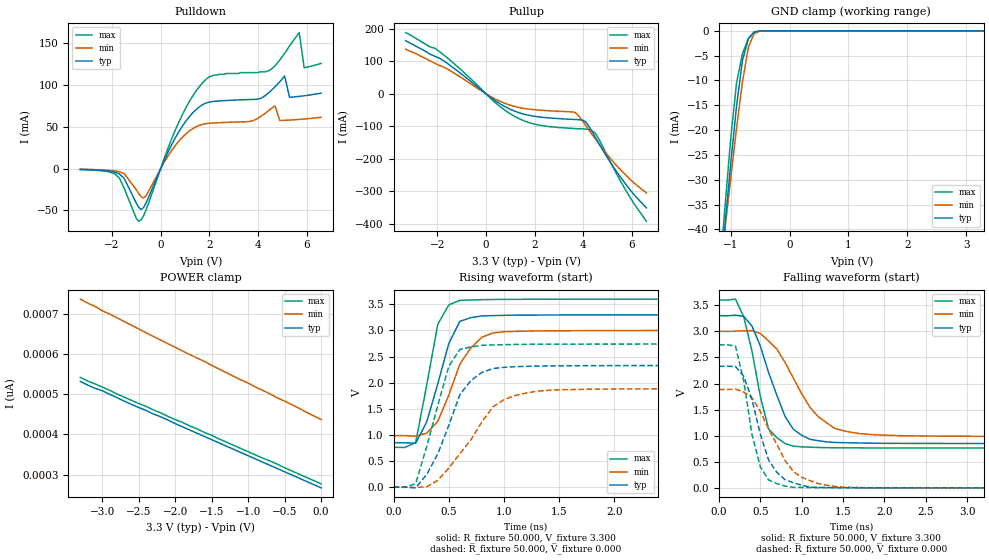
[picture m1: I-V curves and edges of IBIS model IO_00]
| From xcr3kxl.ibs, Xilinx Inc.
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|   Model IO_00
[Model]   IO_00
Model_type   I/O
Polarity   Inverting
Enable   Active-High
Vinl =   0.800V
Vinh =   2.000V
Vmeas =   1.650V
Cref =  50.000pF
Rref =   1.000M
Vref =  0.000V
C_comp   1.250pF   1.000pF   1.500pF
[Temperature Range]   50.000   100.000   0.000
[Voltage Range]   3.300V   3.000V   3.600V
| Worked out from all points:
|   slope of the pulldown table from 0 to 0.495 V, typ, clamps not added: 16 ohm
|   slope of the pullup table from 0 to 0.495 V, typ, clamps not added: 18.3 ohm
|   GND clamp passes 1 mA (typ) near -0.65 V on its own axis
|   rising waveform, R_fixture 50.000, V_fixture 3.300: 20-80 % time 202ps typ, 251ps min, 149ps max; typ from 0.851 V to 3.3 V
|   rising waveform, R_fixture 50.000, V_fixture 0.000: 20-80 % time 278ps typ, 386ps min, 216ps max; typ from 0 V to 2.33 V
|   falling waveform, R_fixture 50.000, V_fixture 3.300: 20-80 % time 334ps typ, 462ps min, 231ps max; typ from 3.3 V to 0.851 V
|   falling waveform, R_fixture 50.000, V_fixture 0.000: 20-80 % time 267ps typ, 385ps min, 199ps max; typ from 2.33 V to 0 V
[Pulldown]
| voltage   I(typ)   I(min)   I(max)
-3.3V     -800uA     -600uA     -1.1mA
-1.7V     -6.1mA     -3.7mA     -11mA
-900mV    -46.35mA   -29.77mA   -62.96mA
-600mV    -41.06mA   -32.32mA   -49.47mA
800mV     46.65mA    34.66mA    59.01mA
1.9V      79mA       54.02mA    108mA
4.5V      92.31mA    70.92mA    118mA
5.1V      111mA      57.94mA    138mA
5.3V      85.46mA    58.26mA    147mA
5.7V      86.62mA    59.04mA    163mA
5.9V      87.32mA    59.5mA     121mA
6.6V      90.4mA     61.49mA    126mA
[Pullup]
| voltage   I(typ)   I(min)   I(max)
-3.3V     163mA      137mA      188mA
-1.9V     109mA      86.62mA    129mA
300mV     -17.18mA   -13mA      -21.73mA
1.2V      -53.91mA   -39.46mA   -70.33mA
2.1V      -70.35mA   -49.69mA   -95.08mA
3.6V      -78.94mA   -56.27mA   -107mA
3.8V      -79.64mA   -66.55mA   -108mA
4.1V      -86.5mA    -97.21mA   -109mA
4.5V      -134mA     -139mA     -121mA
5.5V      -253mA     -231mA     -264mA
6.1V      -311mA     -275mA     -339mA
6.6V      -351mA     -305mA     -392mA
[GND_clamp]
| voltage   I(typ)   I(min)   I(max)
-3.3V     -265mA     -226mA     -304mA
-1.2V     -52.28mA   -50.76mA   -50.82mA
-1.1V     -39.47mA   -40.24mA   -35.9mA
-1V       -26.88mA   -29.77mA   -21.76mA
-900mV    -15.13mA   -19.6mA    -10.45mA
-800mV    -5.967mA   -10.29mA   -4.628mA
-700mV    -1.62mA    -3.333mA   -1.533mA
-600mV    -271uA     -529uA     -194uA
-500mV    -24.86uA   -57.89uA   -10.46uA
-400mV    -1.648uA   -5.395uA   -366nA
3.3V      234pA      465pA      222pA
[POWER_clamp]
| voltage   I(typ)   I(min)   I(max)
-3.3V     532pA      737pA      542pA
-3.2V     523pA      727pA      533pA
-3.1V     515pA      719pA      526pA
-3V       509pA      708pA      518pA
-2.9V     500pA      700pA      510pA
-2.7V     483pA      681pA      493pA
-2.4V     460pA      653pA      470pA
-2.3V     451pA      644pA      461pA
-2.1V     436pA      626pA      445pA
-700mV    323pA      501pA      334pA
-300mV    291pA      465pA      301pA
0V        267pA      437pA      277pA
[Ramp]
| variable   typ   min   max
dV/dt_r   1.397/0.264n   1.131/0.353n   1.644/0.208n
dV/dt_f   1.470/0.303n   1.208/0.452n   1.702/0.213n
R_load = 50.000
[Rising Waveform]
R_fixture = 50.000
V_fixture = 3.300
V_fixture_min = 3.000
V_fixture_max = 3.600
L_fixture = 0.000H
C_fixture = 0.000F
| time   V(typ)   V(min)   V(max)
0s        851mV      986mV      764mV
200ps     843mV      978mV      854mV
300ps     1.249V     1.034V     1.956V
400ps     1.976V     1.257V     3.117V
500ps     2.749V     1.764V     3.49V
600ps     3.175V     2.355V     3.576V
700ps     3.246V     2.667V     3.584V
800ps     3.278V     2.869V     3.589V
1ns       3.29V      2.976V     3.594V
5ns       3.299V     2.999V     3.6V
[Rising Waveform]
R_fixture = 50.000
V_fixture = 0.000
V_fixture_min = 0.000
V_fixture_max = 0.000
L_fixture = 0.000H
C_fixture = 0.000F
| time   V(typ)   V(min)   V(max)
0s        0V         0V         0V
200ps     -13.3mV    -7.882mV   68.17mV
400ps     635mV      130mV      1.565V
500ps     1.184V     365mV      2.313V
600ps     1.771V     640mV      2.636V
700ps     2.04V      905mV      2.685V
900ps     2.271V     1.537V     2.723V
1.1ns     2.307V     1.755V     2.732V
1.3ns     2.318V     1.838V     2.736V
5ns       2.329V     1.885V     2.74V
[Falling Waveform]
R_fixture = 50.000
V_fixture = 3.300
V_fixture_min = 3.000
V_fixture_max = 3.600
L_fixture = 0.000H
C_fixture = 0.000F
| time   V(typ)   V(min)   V(max)
0s        3.3V       3V         3.6V
200ps     3.31V      3.003V     3.617V
300ps     3.286V     3.011V     3.278V
400ps     3.1V       3.012V     2.616V
500ps     2.72V      2.959V     1.754V
600ps     2.211V     2.816V     1.128V
800ps     1.366V     2.4V       849mV
1.1ns     931mV      1.543V     779mV
1.5ns     866mV      1.095V     767mV
5ns       851mV      986mV      764mV
[Falling Waveform]
R_fixture = 50.000
V_fixture = 0.000
V_fixture_min = 0.000
V_fixture_max = 0.000
L_fixture = 0.000H
C_fixture = 0.000F
| time   V(typ)   V(min)   V(max)
0s        2.329V     1.885V     2.74V
200ps     2.326V     1.893V     2.718V
300ps     2.14V      1.836V     2.046V
400ps     1.689V     1.727V     1.021V
500ps     1.033V     1.467V     405mV
600ps     534mV      1.126V     153mV
700ps     296mV      835mV      81.24mV
900ps     96.86mV    312mV      10.43mV
1.4ns     4.624mV    27.43mV    2.201mV
5ns       14.94uV    33.27uV    10.15uV
